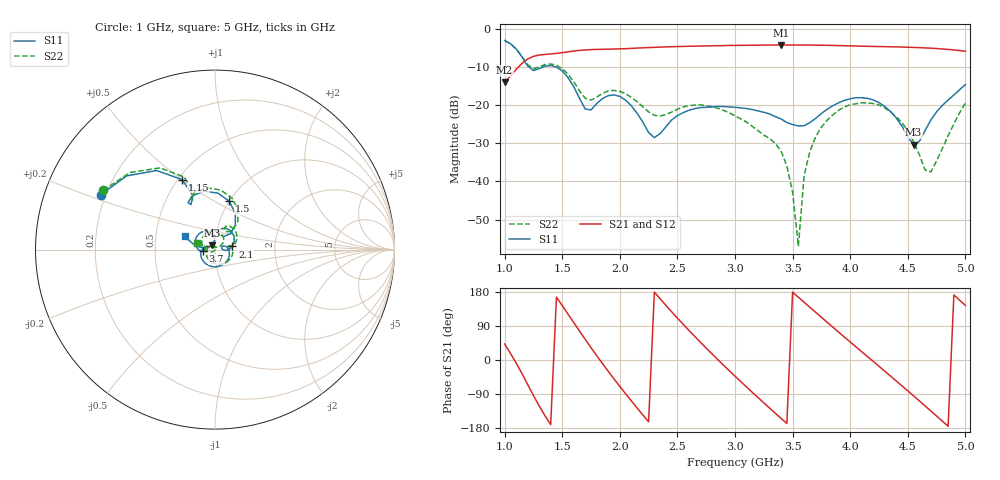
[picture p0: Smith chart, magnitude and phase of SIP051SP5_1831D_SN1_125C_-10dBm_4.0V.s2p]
# GHz  S  dB  R  50
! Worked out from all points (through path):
!   81 points, 1 GHz to 5 GHz, reference 50 ohm
!   highest |S21| = -4.20 dB at 3.4 GHz (marker M1); lowest = -14.0 dB at 1 GHz (marker M2)
!   lowest |S11| = -30.4 dB at 4.55 GHz (marker M3), VSWR 1.06, Z = 48.3 + j2.41 ohm
!   |S11| at or under -10 dB: 1.212 GHz to 1.331 GHz (119.2 MHz wide, 9.37 % of centre); 1.448 GHz to end of sweep
!   |S22| runs from -57.0 to -3.0 dB; largest |S21 - S12| = 0.0021
!   S11 on the Smith chart (normalised r, x): 1 GHz: 0.18, +0.22; 1.15 GHz: 0.52, +0.50; 1.5 GHz: 1.00, +0.59; 2.1 GHz: 1.21, +0.04; 3.7 GHz: 0.87, -0.01; 5 GHz: 0.70, +0.11
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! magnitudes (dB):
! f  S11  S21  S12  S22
! 1 GHz  -3.0  -14.0  -14.0  -3.0
! 1.15 GHz  -7.3  -9.1  -9.1  -7.1
! 1.25 GHz  -10.9  -7.2  -7.2  -10.4
! 1.5 GHz  -11.0  -6.2  -6.2  -10.4
! 1.7 GHz  -21.0  -5.5  -5.5  -18.2
! 1.95 GHz  -17.3  -5.3  -5.3  -16.1
! 2.1 GHz  -20.1  -5.1  -5.1  -18.0
! 2.25 GHz  -27.1  -4.9  -4.9  -21.7
! 2.35 GHz  -27.5  -4.8  -4.7  -22.8
! 2.6 GHz  -21.3  -4.5  -4.5  -20.1
! 3 GHz  -20.5  -4.3  -4.3  -22.8
! 3.4 GHz  -23.6  -4.2  -4.2  -32.0
! 3.5 GHz  -25.1  -4.2  -4.2  -42.8
! 3.55 GHz  -25.4  -4.2  -4.2  -57.0
! 3.6 GHz  -25.4  -4.2  -4.2  -38.4
! 3.7 GHz  -23.4  -4.3  -4.2  -28.3
! 4 GHz  -18.3  -4.4  -4.4  -19.9
! 4.35 GHz  -21.7  -4.7  -4.7  -21.8
! 4.55 GHz  -30.4  -4.8  -4.8  -29.5
! 4.65 GHz  -26.6  -5.0  -5.0  -37.0
! 4.7 GHz  -23.9  -5.0  -5.0  -37.5
! 5 GHz  -14.6  -5.8  -5.9  -19.4
